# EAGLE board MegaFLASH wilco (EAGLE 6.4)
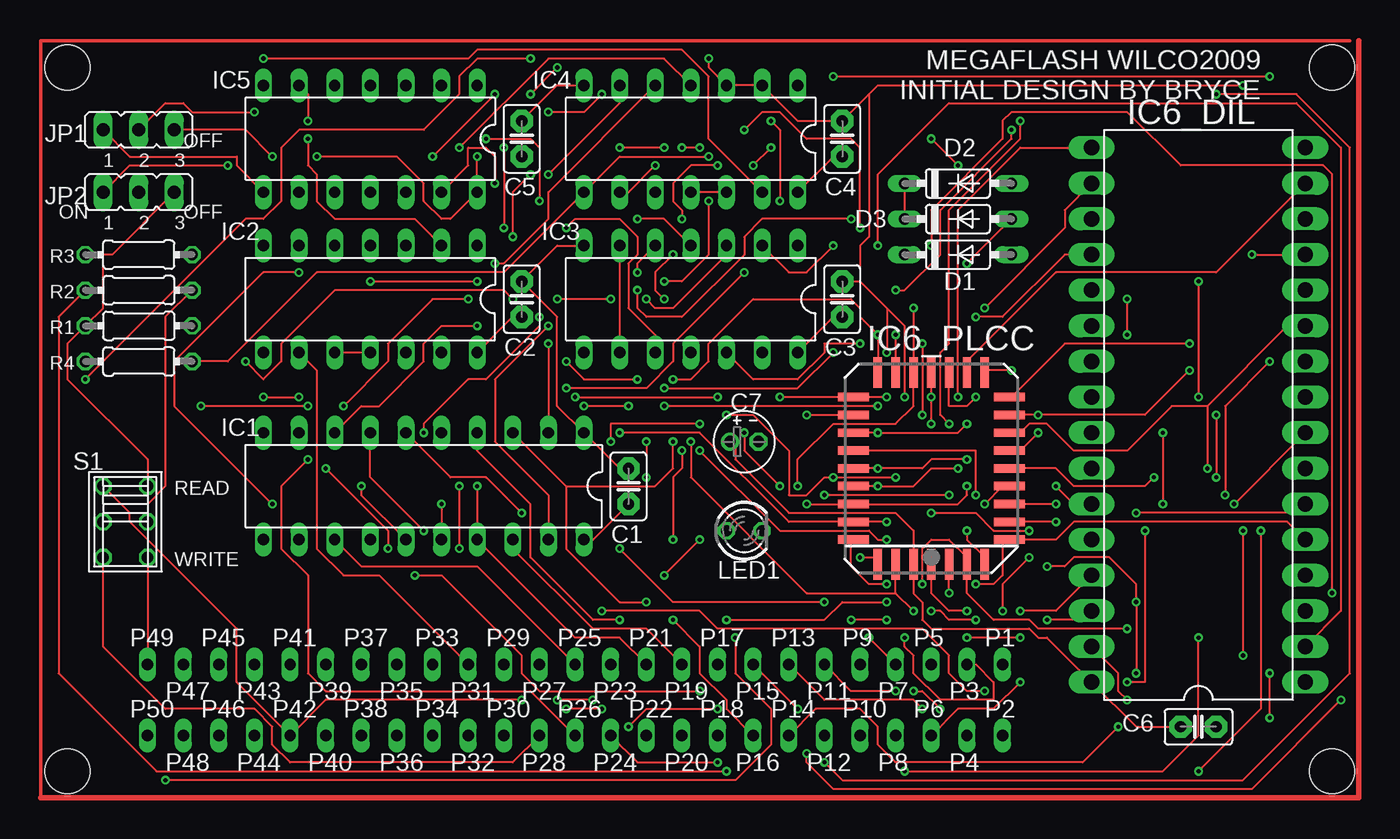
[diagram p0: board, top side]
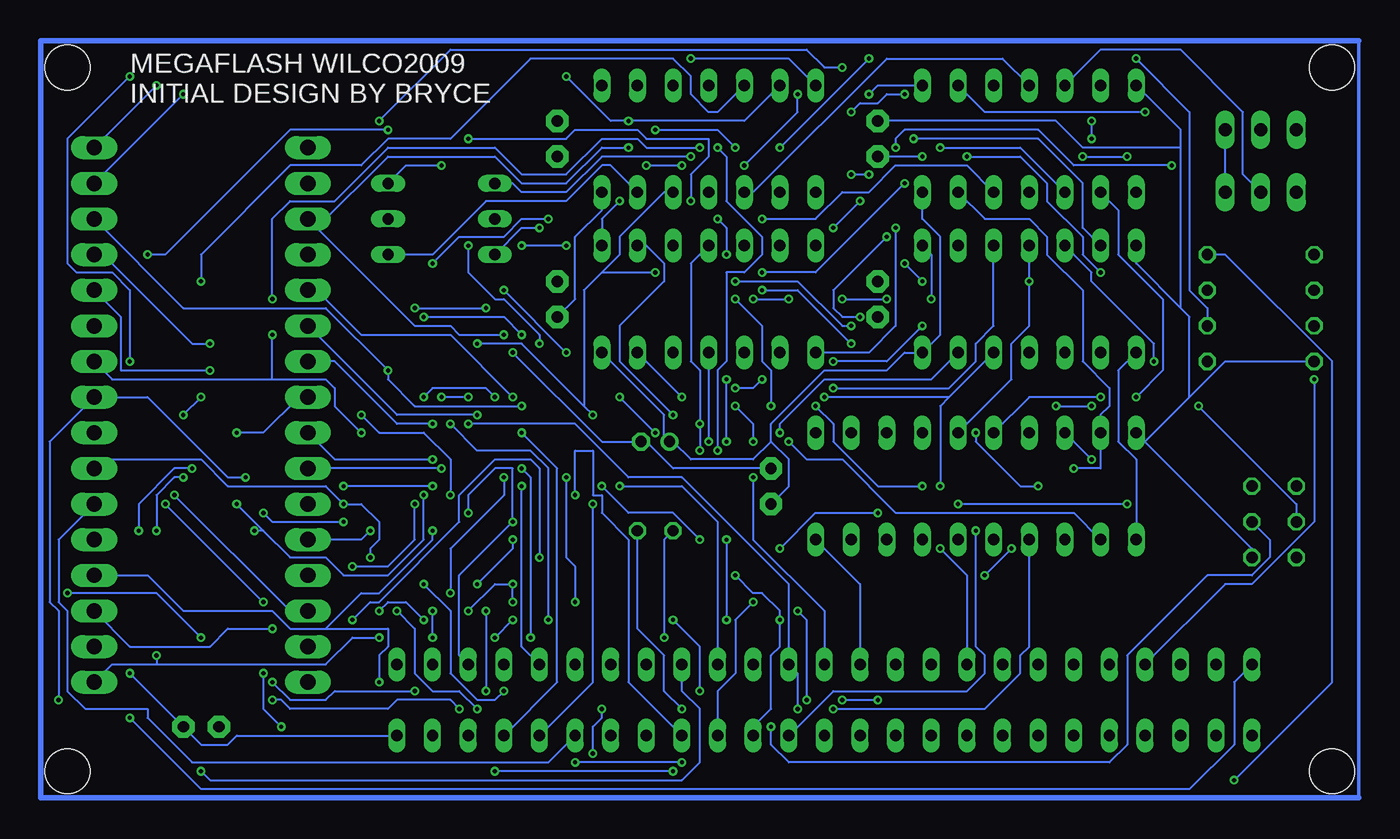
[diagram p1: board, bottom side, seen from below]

No outline drawn. Coordinates in mm, seen from the top.
Copper layers (1*2*15*16): Top 0.035mm / dielectric 0.2mm / Route2 0.0175mm / dielectric 1.1mm / Route15 0.0175mm / dielectric 0.2mm / Bottom 0.035mm
Design rules "SeeedStudio_DRU_no_angle_20130527": minimum track width 6mil, minimum drill 12mil, track to track 6mil, track to pad 6mil, pad to pad 6mil, via to via 6mil, smd to smd 0mil, copper to edge 10mil, drill to drill 10mil, minimum pad ring 6mil, minimum via ring 6mil, stop-mask expansion 2mil, vias tented up to drill 25mil, thermal gap 10mil
Holes 3.2 mm at 1.91,52.07 92.08,52.07 92.08,1.91 1.91,1.91

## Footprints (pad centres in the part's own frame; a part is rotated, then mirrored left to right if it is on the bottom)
C2.5-2 = drill 0.813 pad 1.6 octagon: 1 -1.27,0; 2 1.27,0
E2-4 = drill 0.813 pad 1.27: + -1.016,0 | drill 0.813 pad 1.27 octagon: - 1.016,0
DO35-7 = drill 0.813 long: A 3.81,0; C -3.81,0
CPC_BUS_EXP_BOTTOM = drill 0.813 long: 1 30.48,3.81; 2 30.48,-1.27; 3 27.94,3.81; 4 27.94,-1.27; 5 25.4,3.81; 6 25.4,-1.27; 7 22.86,3.81; 8 22.86,-1.27; 9 20.32,3.81; 10 20.32,-1.27; 11 17.78,3.81; 12 17.78,-1.27; 13 15.24,3.81; 14 15.24,-1.27; 15 12.7,3.81; 16 12.7,-1.27; 17 10.16,3.81; 18 10.16,-1.27; 19 7.62,3.81; 20 7.62,-1.27; 21 5.08,3.81; 22 5.08,-1.27; 23 2.54,3.81; 24 2.54,-1.27; 25 0,3.81; 26 0,-1.27; 27 -2.54,3.81; 28 -2.54,-1.27; 29 -5.08,3.81; 30 -5.08,-1.27; 31 -7.62,3.81; 32 -7.62,-1.27; 33 -10.16,3.81; 34 -10.16,-1.27; 35 -12.7,3.81; 36 -12.7,-1.27; 37 -15.24,3.81; 38 -15.24,-1.27; 39 -17.78,3.81; 40 -17.78,-1.27; 41 -20.32,3.81; 42 -20.32,-1.27; 43 -22.86,3.81; 44 -22.86,-1.27; 45 -25.4,3.81; 46 -25.4,-1.27; 47 -27.94,3.81; 48 -27.94,-1.27; 49 -30.48,3.81; 50 -30.48,-1.27
DIL20 = drill 0.813 long: 1 -11.43,-3.81; 2 -8.89,-3.81; 3 -6.35,-3.81; 4 -3.81,-3.81; 5 -1.27,-3.81; 6 1.27,-3.81; 7 3.81,-3.81; 8 6.35,-3.81; 9 8.89,-3.81; 10 11.43,-3.81; 11 11.43,3.81; 12 8.89,3.81; 13 6.35,3.81; 14 3.81,3.81; 15 1.27,3.81; 16 -1.27,3.81; 17 -3.81,3.81; 18 -6.35,3.81; 19 -8.89,3.81; 20 -11.43,3.81
DIL14 = drill 0.813 long: 1 -7.62,-3.81; 2 -5.08,-3.81; 3 -2.54,-3.81; 4 0,-3.81; 5 2.54,-3.81; 6 5.08,-3.81; 7 7.62,-3.81; 8 7.62,3.81; 9 5.08,3.81; 10 2.54,3.81; 11 0,3.81; 12 -2.54,3.81; 13 -5.08,3.81; 14 -7.62,3.81
DIL32 = drill 1.1 long: 1 -21.59,-8.89; 2 -19.05,-8.89; 3 -16.51,-8.89; 4 -13.97,-8.89; 5 -11.43,-8.89; 6 -8.89,-8.89; 7 -6.35,-8.89; 8 -3.81,-8.89; 9 -1.27,-8.89; 10 1.27,-8.89; 11 3.81,-8.89; 12 6.35,-8.89; 13 8.89,-8.89; 14 11.43,-8.89; 15 13.97,-8.89; 16 16.51,-8.89; 17 16.51,6.35; 18 13.97,6.35; 19 11.43,6.35; 20 8.89,6.35; 21 6.35,6.35; 22 3.81,6.35; 23 1.27,6.35; 24 -1.27,6.35; 25 -3.81,6.35; 26 -6.35,6.35; 27 -8.89,6.35; 28 -11.43,6.35; 29 -13.97,6.35; 30 -16.51,6.35; 31 -19.05,6.35; 32 -21.59,6.35
PLCC32 = smd 2.2 x 0.6: 1 -6.83,0; 2 -6.83,-1.27; 3 -6.83,-2.54; 4 -6.83,-3.81; 14 6.83,-3.81; 15 6.83,-2.54; 16 6.83,-1.27; 17 6.83,0; 18 6.83,1.27; 19 6.83,2.54; 20 6.83,3.81; 30 -6.83,3.81; 31 -6.83,2.54; 32 -6.83,1.27 | smd 0.6 x 2.2: 5 -5.08,-5.56; 6 -3.81,-5.56; 7 -2.54,-5.56; 8 -1.27,-5.56; 9 0,-5.56; 10 1.27,-5.56; 11 2.54,-5.56; 12 3.81,-5.56; 13 5.08,-5.56; 21 5.08,5.56; 22 3.81,5.56; 23 2.54,5.56; 24 1.27,5.56; 25 0,5.56; 26 -1.27,5.56; 27 -2.54,5.56; 28 -3.81,5.56; 29 -5.08,5.56
JP2 = drill 0.914 long: 1 -2.54,0; 2 0,0; 3 2.54,0
LED3MM = drill 0.813 octagon: A -1.27,0; K 1.27,0
0204/7 = drill 0.813 octagon: 1 -3.81,0; 2 3.81,0
2P2T-FINO = drill 0.813 octagon: 1 -2.54,-1.27; 2 0,-1.27; 3 2.54,-1.27; 4 -2.54,1.905; 5 0,1.905; 6 2.54,1.905

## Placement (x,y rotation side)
C1  100nF  [C2.5-2]  41.91,22.23 90 top
C2  100nF  [C2.5-2]  34.29,35.56 90 top
C3  100nF  [C2.5-2]  57.15,35.56 90 top
C4  100nF  [C2.5-2]  57.15,46.99 90 top
C5  100nF  [C2.5-2]  34.29,46.99 90 top
C6  100nF  [C2.5-2]  82.55,5.08 0 top
C7  100microF  [E2-4]  50.16,25.4 0 top
D1  1N4148DO35-7  [DO35-7]  65.41,38.73 0 top
D2  1N4148DO35-7  [DO35-7]  65.41,43.81 0 top
D3  1N4148DO35-7  [DO35-7]  65.41,41.27 0 top
EC1  CPC_BUS_EXPBOTTOM  [CPC_BUS_EXP_BOTTOM]  38.1,5.71 0 top
IC1  74LS374N  [DIL20]  27.3,22.23 180 top
IC2  74LS32N  [DIL14]  23.5,35.56 180 top
IC3  74LS32N  [DIL14]  46.35,35.56 180 top
IC4  74LS02N  [DIL14]  46.35,46.99 180 top
IC5  74LS20N  [DIL14]  23.5,46.99 180 top
IC6_DIL  29C040DIL32  [DIL32]  81.28,29.84 90 top
IC6_PLCC  29C040PLCC32  [PLCC32]  63.5,23.5 90 top
JP1  ROM 7  [JP2]  6.99,47.62 0 top
JP2  ROM 0  [JP2]  6.99,43.18 0 top
LED1  TLLR4400  [LED3MM]  50.16,19.05 0 top
R1  1K  [0204/7]  6.99,33.66 180 top
R2  220R  [0204/7]  6.99,36.2 180 top
R3  1K  [0204/7]  6.99,38.73 0 top
R4  1K  [0204/7]  6.99,31.11 0 top
S1  DPDT  [2P2T-FINO]  5.71,19.68 270 top

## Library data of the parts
C1-C6 = capacitor-wima
C7 = resistor
D1-D3 = diode
EC1 IC6_DIL IC6_PLCC S1 = Mio
IC1-IC5 = 74xx-eu
JP1 JP2 = jumper
LED1 = led; MF: VISHAY SEMICONDUCTOR; OC_FARNELL: 1612437
R1-R4 = eagle-ltspice; SPICEMODEL: NONE; SPICEPREFIX: R

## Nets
GND: C1.2 C2.2 C3.2 C4.2 C5.2 C6.2 C7.- EC1.2 EC1.49 IC1.1 IC1.10 IC2.7 IC3.7 IC4.2 IC4.3 IC4.7 IC5.7 IC6_DIL.16 IC6_PLCC.16 R4.1 S1.6
N$1: EC1.3 IC5.1
N$2: EC1.12 IC6_DIL.6 IC6_PLCC.6
N$3: EC1.31 IC2.9
N$5: EC1.7 IC6_DIL.25 IC6_PLCC.25
N$6: IC1.9 IC3.5 IC5.13 IC6_DIL.29 IC6_PLCC.29
N$7: IC1.12 IC3.4 IC5.12 IC6_DIL.3 IC6_PLCC.3
N$8: EC1.9 IC6_DIL.26 IC6_PLCC.26
N$9: EC1.11 IC6_DIL.5 IC6_PLCC.5
N$10: EC1.13 IC6_DIL.7 IC6_PLCC.7
N$11: EC1.15 IC6_DIL.9 IC6_PLCC.9
N$12: EC1.17 IC6_DIL.11 IC6_PLCC.11
N$13: IC1.6 IC3.2 IC5.9 IC6_DIL.2 IC6_PLCC.2
N$14: EC1.6 IC6_DIL.4 IC6_PLCC.4
N$15: EC1.8 IC6_DIL.23 IC6_PLCC.23
N$16: EC1.10 IC6_DIL.27 IC6_PLCC.27
N$17: EC1.14 IC6_DIL.8 IC6_PLCC.8
N$18: EC1.16 IC6_DIL.10 IC6_PLCC.10
N$19: EC1.18 IC6_DIL.12 IC6_PLCC.12
N$20: EC1.26 IC1.8 IC6_DIL.13 IC6_PLCC.13
N$21: EC1.24 IC1.7 IC6_DIL.15 IC6_PLCC.15
N$22: EC1.22 IC1.4 IC6_DIL.18 IC6_PLCC.18
N$23: EC1.20 IC1.3 IC6_DIL.20 IC6_PLCC.20
N$24: EC1.25 IC1.13 IC6_DIL.14 IC6_PLCC.14
N$25: EC1.23 IC1.14 IC6_DIL.17 IC6_PLCC.17
N$26: EC1.21 IC1.17 IC6_DIL.19 IC6_PLCC.19
N$27: EC1.19 IC1.18 IC6_DIL.21 IC6_PLCC.21
N$28: IC1.15 IC3.1 IC4.6 IC6_DIL.30 IC6_PLCC.30
N$29: IC1.5 IC2.4 IC4.5 IC6_DIL.1 IC6_PLCC.1
N$30: IC2.3 IC4.11 IC4.12 IC6_DIL.22 IC6_PLCC.22
N$33: EC1.42 IC6_DIL.24 IC6_PLCC.24 S1.1
N$34: IC3.11 IC6_DIL.31 IC6_PLCC.31
N$35: D1.C EC1.43
N$36: EC1.28 S1.3
N$37: D1.A IC4.13 R1.1
N$38: LED1.A R3.2
N$39: LED1.K R2.1 S1.5
N$40: IC3.12 R2.2
N$41: IC2.5 IC3.3
N$42: EC1.33 IC2.12 IC3.13
N$43: IC3.6 IC3.9
N$44: IC2.6 IC3.10
N$45: IC1.11 IC2.8
N$46: IC2.1 S1.2
N$47: IC2.2 IC5.6
N$48: IC2.10 IC2.11
N$49: IC4.4 IC5.10
N$50: IC4.10 IC5.4
N$51: IC5.8 JP1.1
N$52: IC5.5 JP2.2
N$53: IC5.2 JP1.2
N$54: IC3.8 JP2.1
N$55: D2.A IC1.19
N$56: IC1.16 IC4.9
N$57: D2.C D3.C IC4.8 R4.2
N$58: EC1.5 IC2.13 IC6_DIL.28 IC6_PLCC.28
N$59: D3.A IC1.2
VCC: C1.1 C2.1 C3.1 C4.1 C5.1 C6.1 C7.+ EC1.27 IC1.20 IC2.14 IC3.14 IC4.14 IC5.14 IC6_DIL.32 IC6_PLCC.32 JP1.3 JP2.3 R1.2 R3.1 S1.4

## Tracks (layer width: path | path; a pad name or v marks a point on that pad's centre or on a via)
GND  (via drill 0.3)
  Top 0.152: IC3.7 36.83,39.37 C2.2 36.83,34.29 36.83,27.94 IC1.1 41.27,23.5 C1.2 | IC6_PLCC.16 64.77,27.94 66.04,27.94 v66.67,28.57 | v61.59,28.57 61.59,33.66 60.33,34.92 | 58.42,36.83 60.33,34.92 | C3.2 58.42,36.83 | v85.72,50.8 59.69,50.8 59.05,50.16 | 59.05,50.16 C4.2 53.98,48.26 IC4.2 IC4.3 47.62,52.07 v47.62,52.7 | 58.42,36.83 58.42,39.37 59.05,40.01 59.05,50.16 | 60.33,34.92 v60.33,31.75 | IC4.7 36.83,50.8 C5.2 | S1.6 EC1.49 | v87.63,5.71 v87.63,8.89
  Bottom 0.152: C1.2 48.9,23.5 50.8,25.4 C7.- 53.98,25.4 v60.33,31.75 | v66.67,28.57 66.04,29.21 62.23,29.21 v61.59,28.57 | v85.72,50.8 IC6_DIL.16 | EC1.2 80.01,4.45 80.64,3.81 82.55,3.81 C6.2 v87.63,8.89 | 15.24,25.4 7.62,17.78 S1.6 | 15.24,25.4 IC1.10 | R4.1 9.53,31.11 12.06,28.57 | 15.24,25.4 12.06,28.57 | IC2.7 15.88,38.1 12.7,34.92 | 12.7,34.92 12.06,34.29 12.06,28.57 | IC5.7 12.7,47.62 12.7,46.35 | 12.7,34.92 12.7,46.35 | C5.2 21.59,48.26 19.68,46.35 12.7,46.35 | v87.63,5.71 82.55,0.64 12.06,0.64 8.89,3.81 8.89,8.26 EC1.49 | v47.62,52.7 40.64,52.7 IC4.7
N$1  (via drill 0.3)
  Top 0.152: v36.83,52.07 v34.92,50.16 | v69.85,48.26 69.85,46.99 64.77,41.91 64.77,32.38 64.14,31.75 64.14,27.3 v64.77,26.67 | v60.33,12.7 v57.78,12.7 | v61.59,11.43 61.59,10.79 62.23,10.16 62.23,8.89 64.14,6.99 67.94,6.99 67.94,8.26 66.67,9.53 EC1.3
  Bottom 0.152: IC5.1 34.29,50.8 v34.92,50.16 | v36.83,52.07 38.1,52.07 39.37,53.34 64.77,53.34 v69.85,48.26 | v64.77,26.67 62.87,24.77 59.05,24.77 57.78,23.5 v57.78,12.7 | v61.59,11.43 v60.33,12.7
N$2  (via drill 0.3)
  Top 0.152: v72.39,19.68 IC6_PLCC.6 | v78.11,20.32 89.53,20.32 IC6_DIL.6
  Bottom 0.152: v72.39,19.68 77.47,19.68 v78.11,20.32 | EC1.12 57.78,2.54 83.19,2.54 86.36,5.71 86.36,6.35 90.81,6.35 92.08,7.62 92.08,13.34 92.71,13.97 92.71,18.41 IC6_DIL.6
N$3
  Top 0.152: EC1.31 24.13,15.88 21.59,15.88 19.68,17.78 19.68,30.48 IC2.9
N$5  (via drill 0.3)
  Top 0.152: IC6_PLCC.25 v59.69,23.5 62.87,23.5 63.5,24.13 v66.04,24.13 | v59.05,11.43 EC1.7
  Bottom 0.152: v66.04,24.13 73.03,24.13 IC6_DIL.25 | v59.05,11.43 59.05,22.86 v59.69,23.5
N$6  (via drill 0.3)
  Top 0.152: v60.33,15.24 59.05,15.24 57.78,16.51 57.78,18.41 IC6_PLCC.29 | v63.5,13.34 64.14,13.34 64.77,12.7 v66.67,12.7 | v69.85,13.34 72.39,13.34 IC6_DIL.29 | IC3.5 42.55,38.1 v42.55,37.47 | v32.38,43.81 32.38,45.72 31.75,46.35 30.48,46.35 30.48,45.09 IC5.13 | v60.33,13.97 57.15,13.97 55.88,12.7 v48.9,12.7 | v46.99,7.62 35.56,7.62 34.29,8.89 34.29,10.16 28.57,15.88 v26.67,15.88 | v24.77,17.78 24.77,19.05 v20.32,23.5
  Bottom 0.152: v63.5,13.34 61.59,15.24 v60.33,15.24 v60.33,13.97 | v66.67,12.7 67.94,13.97 69.22,13.97 v69.85,13.34 | IC5.13 26.67,41.27 23.5,41.27 22.23,40.01 22.23,38.73 19.68,36.2 19.68,31.11 17.78,29.21 17.78,27.94 18.41,27.3 IC1.9 18.41,23.5 v20.32,23.5 | v42.55,37.47 38.73,37.47 v32.38,43.81 | v48.9,12.7 46.99,10.79 v46.99,7.62 | v24.77,17.78 v26.67,15.88
N$7  (via drill 0.3)
  Top 0.152: v77.47,12.06 71.12,12.06 70.48,12.7 67.94,12.7 66.04,14.61 IC6_PLCC.3 66.04,17.14 64.77,18.41 63.5,18.41 62.87,17.78 v62.87,15.24 | v40.64,25.4 40.64,26.67 v46.99,26.67 | v42.55,41.27 44.45,41.27 IC3.4 | v60.33,18.41 59.69,18.41 59.05,19.05 52.7,19.05 v46.99,24.77
  Bottom 0.152: v77.47,12.06 80.64,12.06 81.92,10.79 87.63,10.79 IC6_DIL.3 | IC1.12 20.32,20.32 33.02,20.32 36.83,24.13 39.37,24.13 v40.64,25.4 | IC3.4 47.62,38.1 47.62,31.11 46.99,30.48 v46.99,26.67 v46.99,24.77 | IC5.12 27.94,45.09 33.02,45.09 34.92,43.18 36.83,43.18 38.73,41.27 v42.55,41.27 | v62.87,15.24 60.33,17.78 v60.33,18.41
N$8  (via drill 0.3)
  Top 0.152: IC6_PLCC.26 v59.69,22.23 62.23,22.23 63.5,23.5 v65.41,23.5
  Bottom 0.152: v59.69,22.23 59.69,10.79 EC1.9 | v65.41,23.5 IC6_DIL.26
N$9  (via drill 0.3)
  Top 0.152: IC6_DIL.5 88.9,19.68 73.66,19.68 72.39,18.41 IC6_PLCC.5 68.58,18.41 68.58,15.88 67.94,15.24 v66.67,15.24 | EC1.11 57.78,7.62 v60.96,7.62
  Bottom 0.152: v60.96,7.62 61.59,6.99 62.87,6.99 64.77,8.89 64.77,13.34 v66.67,15.24
N$10  (via drill 0.3)
  Top 0.152: v72.39,20.95 IC6_PLCC.7 | EC1.13 55.88,6.99 62.23,6.99 v62.87,6.35 | v68.58,13.34 68.58,15.24 v70.48,17.14
  Bottom 0.152: IC6_DIL.7 89.53,24.13 82.55,24.13 80.64,22.23 73.66,22.23 v72.39,20.95 71.12,20.95 69.85,19.68 69.85,18.41 70.48,17.78 v70.48,17.14 | v62.87,6.35 64.14,7.62 66.04,7.62 67.31,8.89 67.31,12.06 v68.58,13.34
N$11  (via drill 0.3)
  Top 0.152: IC6_PLCC.9 72.39,23.5 73.66,22.23 78.74,22.23 v79.38,22.86 | v53.98,6.35 EC1.15 | v54.61,3.17 54.61,2.54 56.52,0.64 86.36,0.64 v92.71,6.99
  Bottom 0.152: v79.38,22.86 80.64,22.86 86.36,28.57 IC6_DIL.9 93.34,25.4 93.34,13.97 92.71,13.34 v92.71,6.99 | v53.98,6.35 53.98,5.71 54.61,5.08 v54.61,3.17
N$12  (via drill 0.3)
  Top 0.152: IC6_PLCC.11 69.85,26.04 70.48,26.67 71.75,26.67 73.66,24.77 77.47,24.77 80.64,27.94 83.19,27.94 | 83.19,27.94 88.9,33.66 IC6_DIL.11 | v82.55,1.91 87,6.35 v87,19.05 | 83.19,27.94 v83.19,23.5
  Bottom 0.152: EC1.17 48.26,7.62 46.99,6.35 46.99,2.54 48.26,1.27 81.92,1.27 v82.55,1.91 | v87,19.05 87,20.95 84.45,23.5 v83.19,23.5
N$13  (via drill 0.3)
  Top 0.152: v15.88,28.57 v18.41,28.57 | v64.77,14.61 IC6_PLCC.2 | v60.96,22.86 v56.52,22.86 55.88,22.86 54.61,21.59 53.34,21.59 53.34,24.77 50.8,27.3 v48.9,27.3 | IC6_DIL.2 92.71,13.34 92.71,46.35 89.53,49.53 64.77,49.53 59.69,44.45 v59.69,39.37 | v56.52,39.37 54.61,37.47 53.34,37.47 IC3.2 | IC1.6 29.21,22.86 31.75,22.86 v34.29,20.32 | v41.27,17.78 45.09,13.97 v55.88,13.97
  Bottom 0.152: IC1.6 23.5,28.57 v18.41,28.57 | v15.88,28.57 13.97,30.48 13.97,35.56 17.14,38.73 17.14,41.91 IC5.9 | v64.77,14.61 64.77,17.78 60.96,21.59 v60.96,22.86 | v48.9,27.3 52.7,31.11 52.7,33.66 49.53,36.83 49.53,38.1 50.8,39.37 IC3.2 | v56.52,39.37 v59.69,39.37 | v34.29,20.32 38.73,20.32 v41.27,17.78 | v55.88,13.97 55.88,16.51 56.52,17.14 v56.52,22.86
N$14  (via drill 0.3)
  Top 0.152: v66.04,19.05 66.04,18.41 67.31,17.14 IC6_PLCC.4 | EC1.6 65.41,6.35 67.94,6.35 v69.85,8.26
  Bottom 0.152: v66.04,19.05 66.04,18.41 69.85,14.61 71.12,14.61 73.66,12.06 | 73.66,12.06 76.2,12.06 77.47,13.34 83.82,13.34 86.36,15.88 IC6_DIL.4 | v69.85,8.26 69.85,10.16 69.22,10.79 69.22,12.06 73.66,12.06
N$15  (via drill 0.3)
  Top 0.152: IC6_PLCC.23 v59.69,26.04 65.41,26.04 v66.04,26.67
  Bottom 0.152: v59.69,26.04 57.15,23.5 57.15,8.26 EC1.8 | IC6_DIL.23 73.03,31.11 68.58,26.67 v66.04,26.67
N$16  (via drill 0.3)
  Top 0.152: v54.61,20.95 IC6_PLCC.27 65.41,20.95 66.04,21.59 v66.04,22.23 | IC6_DIL.27 73.66,20.95 v72.39,22.23
  Bottom 0.152: v54.61,20.95 54.61,8.26 EC1.10 | v66.04,22.23 v72.39,22.23
N$17  (via drill 0.3)
  Top 0.152: v67.31,20.95 68.58,22.23 IC6_PLCC.8 | v71.75,16.51 73.03,16.51 73.66,17.14 76.2,17.14 78.11,15.24 v78.11,13.97 v78.11,8.89 | IC6_DIL.8 v85.09,20.95 | EC1.14 55.24,6.35 58.42,6.35 59.69,5.08 59.69,3.81 60.96,2.54 74.3,2.54 v76.83,5.08
  Bottom 0.152: v67.31,20.95 67.31,18.41 69.22,16.51 v71.75,16.51 | v85.09,20.95 v78.11,13.97 | v76.83,5.08 78.11,6.35 v78.11,8.89
N$18  (via drill 0.3)
  Top 0.152: IC6_PLCC.10 69.85,24.77 v71.12,26.04 | EC1.16 48.9,6.35 48.9,6.99 46.99,8.89 46.99,10.79 v45.09,12.7 | v45.09,18.41 45.09,22.86 45.72,23.5 v45.72,24.77 | v46.99,46.35 v45.72,46.35 | v77.47,33.02 v77.47,35.56
  Bottom 0.152: v71.12,26.04 73.03,27.94 73.03,29.21 73.66,29.84 77.47,29.84 | 77.47,29.84 88.9,29.84 IC6_DIL.10 | v45.09,18.41 v45.09,12.7 | v45.72,24.77 45.72,30.48 45.09,31.11 45.09,37.47 43.81,37.47 42.55,38.73 42.55,40.01 45.09,42.55 45.09,45.72 v45.72,46.35 | v46.99,46.35 50.8,46.35 51.44,46.99 53.98,46.99 56.52,44.45 59.69,44.45 61.59,46.35 69.22,46.35 73.03,42.55 76.2,42.55 77.47,41.27 v77.47,35.56 | 77.47,29.84 v77.47,33.02
N$19  (via drill 0.3)
  Top 0.152: IC6_PLCC.12 v71.12,27.3 78.74,27.3 v81.92,30.48 | v64.77,21.59 v55.88,21.59
  Bottom 0.152: v81.92,30.48 88.27,30.48 88.27,34.29 IC6_DIL.12 | EC1.18 52.07,8.26 52.07,18.41 53.98,20.32 53.98,21.59 54.61,21.59 54.61,24.77 55.88,24.77 v55.88,21.59 | v64.77,21.59 64.77,24.13 66.67,26.04 69.85,26.04 v71.12,27.3
N$20  (via drill 0.3)
  Top 0.152: v81.92,32.38 73.03,32.38 69.22,28.57 IC6_PLCC.13 | EC1.26 34.92,7.62 20.32,7.62 19.05,8.89 19.05,15.88 17.14,17.78 17.14,22.23 v19.05,24.13 | v86.36,38.73 IC6_DIL.13 | v69.22,47.62 69.22,46.99 64.14,41.91 64.14,38.73 61.59,36.2 v60.96,36.2 | v56.52,31.75 53.98,29.21 v44.45,29.21 | v42.55,29.84 38.73,29.84 v37.47,31.11 | v31.11,33.66 28.57,33.66 27.3,32.38 27.3,31.11 24.13,27.94 22.86,27.94 IC1.8
  Bottom 0.152: v81.92,32.38 83.19,32.38 89.53,38.73 IC6_DIL.13 | IC1.8 v19.05,24.13 | v86.36,38.73 85.09,38.73 76.2,47.62 v69.22,47.62 | v56.52,31.75 v60.96,36.2 | v44.45,29.21 43.18,29.21 v42.55,29.84 | v37.47,31.11 33.66,31.11 v31.11,33.66
N$21  (via drill 0.3)
  Top 0.152: IC6_PLCC.15 66.04,31.11 72.39,37.47 83.82,37.47 IC6_DIL.15 | IC1.7 23.5,22.86 v27.3,19.05 | v83.82,50.16 89.53,50.16 93.34,46.35 93.34,8.89 85.72,1.27 57.15,1.27 v55.88,2.54 | v48.26,2.54 42.55,2.54 EC1.24
  Bottom 0.152: v27.3,19.05 27.3,10.79 26.67,10.16 26.67,8.89 27.94,7.62 37.47,7.62 EC1.24 | v83.82,50.16 IC6_DIL.15 | v48.26,2.54 v55.88,2.54
N$22  (via drill 0.3)
  Top 0.152: v62.23,34.92 IC6_PLCC.18 62.23,27.94 60.96,26.67 56.52,26.67 53.98,24.13 v53.98,22.23 | v67.31,34.92 73.03,40.64 73.03,41.91 IC6_DIL.18 | IC1.4 31.11,24.77 34.92,20.95 34.92,17.14 39.37,12.7 v41.27,12.7 | v44.45,15.88 v46.99,18.41
  Bottom 0.152: v67.31,34.92 v62.23,34.92 | EC1.22 43.18,5.08 41.91,6.35 41.91,10.16 41.27,10.79 v41.27,12.7 41.27,13.34 42.55,14.61 43.18,14.61 v44.45,15.88 | v53.98,22.23 52.07,20.32 48.9,20.32 v46.99,18.41
N$23  (via drill 0.3)
  Top 0.152: IC6_PLCC.20 v59.69,33.02 58.42,34.29 58.42,34.92 57.78,35.56 50.8,35.56 47.62,32.38 47.62,31.11 46.35,29.84 v45.09,29.84 | v66.67,34.29 68.58,34.29 73.03,38.73 IC6_DIL.20 | v43.18,13.97 41.27,13.97 37.47,17.78 37.47,22.23 | IC1.3 37.47,22.23 | v45.09,25.4 45.09,23.5 43.81,22.23 37.47,22.23
  Bottom 0.152: v59.69,33.02 60.96,34.29 v66.67,34.29 | EC1.20 45.72,7.62 44.45,8.89 44.45,12.7 v43.18,13.97 | v45.09,25.4 v45.09,29.84
N$24  (via drill 0.3)
  Top 0.152: EC1.25 31.11,16.51 22.86,16.51 IC1.13 | v69.22,30.48 67.31,30.48 IC6_PLCC.14 | v43.18,25.4 v43.18,22.86 | v59.69,27.94 v44.45,27.94
  Bottom 0.152: IC6_DIL.14 83.82,34.92 73.66,34.92 v69.22,30.48 69.22,29.84 67.31,27.94 v59.69,27.94 | EC1.25 38.1,13.34 43.18,18.41 v43.18,22.86 | v43.18,25.4 43.18,26.67 v44.45,27.94
N$25  (via drill 0.3)
  Top 0.152: v63.5,26.67 v63.5,28.57 IC6_PLCC.17 | v40.01,6.35 v37.47,6.35 | IC6_DIL.17 69.85,46.35 65.41,41.91 v65.41,28.57
  Bottom 0.152: v63.5,26.67 55.88,26.67 52.07,22.86 48.26,22.86 40.64,15.24 EC1.23 40.01,8.89 v40.01,6.35 | IC1.14 23.5,10.79 24.13,10.16 24.13,8.89 26.67,6.35 v37.47,6.35 | v63.5,28.57 v65.41,28.57
N$26  (via drill 0.3)
  Top 0.152: EC1.21 41.27,11.43 38.1,11.43 IC1.17 v31.11,22.23 | v60.96,33.02 IC6_PLCC.19 | v41.91,27.94 v38.73,27.94 | v44.45,35.56 43.81,36.2 43.81,37.47 v45.09,38.73 | v45.72,41.27 45.72,41.91 45.09,42.55 45.09,43.81 46.35,45.09 v48.26,45.09 | v52.07,46.35 v50.8,45.09
  Bottom 0.152: v60.96,33.02 64.14,33.02 64.77,33.66 67.31,33.66 74.3,40.64 | v31.11,22.23 34.29,22.23 37.47,25.4 37.47,26.67 v38.73,27.94 | v41.91,27.94 41.91,30.48 42.55,31.11 42.55,33.66 v44.45,35.56 | v45.09,38.73 45.09,40.64 v45.72,41.27 | v50.8,45.09 v48.26,45.09 | v52.07,46.35 53.98,46.35 56.52,43.81 59.69,43.81 61.59,45.72 69.22,45.72 74.3,40.64 | 74.3,40.64 IC6_DIL.19
N$27  (via drill 0.3)
  Top 0.152: IC1.18 33.66,17.78 39.37,12.06 43.18,12.06 EC1.19 | v60.33,28.57 IC6_PLCC.21 v52.7,28.57 | v52.7,22.23 50.16,24.77 v50.16,26.04
  Bottom 0.152: v60.33,28.57 64.77,33.02 71.12,33.02 74.3,36.2 IC6_DIL.21 | EC1.19 45.72,19.68 48.26,22.23 v52.7,22.23 | v52.7,28.57 v50.16,26.04
N$28  (via drill 0.3)
  Top 0.152: v58.42,17.14 59.69,17.14 IC6_PLCC.30 | v71.75,12.7 74.3,12.7 IC6_DIL.30 | IC1.15 22.86,21.59 v22.86,22.23 | v27.3,26.04 27.3,26.67 30.48,29.84 31.75,29.84 35.56,33.66 v35.56,34.29 | v33.66,40.01 33.66,43.18 v34.92,44.45 | v36.2,44.45 41.27,49.53 IC4.6 | v52.7,42.55 52.7,47.62 v52.07,48.26 | v84.45,21.59 84.45,27.94 v87.63,31.11 | v56.52,51.44 v87.63,51.44
  Bottom 0.152: v58.42,17.14 58.42,23.5 59.05,24.13 61.59,24.13 64.14,21.59 64.14,19.68 69.85,13.97 70.48,13.97 v71.75,12.7 | v22.86,22.23 24.13,22.23 27.3,25.4 v27.3,26.04 | v35.56,34.29 36.83,34.29 37.47,34.92 37.47,36.2 v33.66,40.01 | v36.2,44.45 v34.92,44.45 | IC3.1 53.98,41.27 v52.7,42.55 | IC4.6 43.81,48.26 v52.07,48.26 53.34,48.26 v56.52,51.44 | IC6_DIL.30 76.2,13.34 v84.45,21.59 | v87.63,31.11 87.63,36.2 88.9,37.47 91.44,37.47 92.08,38.1 92.08,46.99 v87.63,51.44
N$29  (via drill 0.3)
  Top 0.152: IC6_PLCC.1 63.5,14.61 64.77,13.34 v66.04,13.34 | v69.85,11.43 v66.04,11.43 | IC4.5 36.2,43.18 36.2,41.27 33.02,38.1 v32.38,38.1 | v23.5,36.83 v31.11,36.83 | v85.72,19.05 v85.72,10.16 | v83.82,27.3 v83.82,22.86 | v82.55,36.83 v82.55,28.57
  Bottom 0.152: v66.04,11.43 v66.04,13.34 | v69.85,11.43 71.75,11.43 73.66,9.53 85.72,9.53 | 85.72,9.53 88.9,9.53 IC6_DIL.1 | IC2.4 v23.5,36.83 23.5,33.66 24.77,32.38 24.77,29.84 IC1.5 | v31.11,36.83 v32.38,38.1 | v85.72,10.16 85.72,9.53 | v85.72,19.05 85.72,21.59 84.45,22.86 v83.82,22.86 | v82.55,28.57 v83.82,27.3 | v82.55,36.83 82.55,38.73 76.2,45.09 71.12,45.09 69.22,46.99 64.77,46.99 59.05,52.7 48.9,52.7 47.62,51.44 47.62,50.16 46.35,48.9 45.72,48.9 IC4.5
N$30  (via drill 0.3)
  Top 0.152: v54.61,27.3 IC6_PLCC.22 | v37.47,29.21 43.18,29.21 45.09,31.11 45.09,32.38 v50.16,37.47 | IC4.12 IC4.11 | v62.87,32.38 v62.87,27.3
  Bottom 0.152: 55.24,27.94 v54.61,27.3 | 55.24,27.94 55.24,36.2 53.98,37.47 | 53.98,37.47 52.7,38.73 52.7,40.01 49.53,43.18 IC4.12 | IC2.3 26.04,33.66 27.3,32.38 27.3,31.11 29.21,29.21 v37.47,29.21 | 53.98,37.47 v50.16,37.47 | IC6_DIL.22 68.58,27.3 v62.87,27.3 | v62.87,32.38 59.69,32.38 55.24,27.94
N$31
  Bottom 0.254: 0,0 0,53.98
  Bottom 0.406: 0,53.98 93.98,53.98 93.98,0 0,0
N$32
  Top 0.254: 93.34,53.98 0,53.98 0,0
  Top 0.406: 0,0 93.98,0 93.98,53.98
N$33  (via drill 0.3)
  Top 0.152: S1.1 6.35,20.32 6.35,19.68 13.97,12.06 13.97,8.26 EC1.42 20.32,6.99 v34.29,6.99 | IC6_PLCC.24 66.67,24.77 v66.67,21.59 | v80.01,26.04 v80.01,20.95 | v39.37,6.99 v36.83,6.99 | v40.01,13.34 46.99,13.34 48.26,12.06 62.87,12.06 64.77,10.16 64.77,8.89 66.04,7.62 v67.31,7.62 | v77.47,8.26 78.74,8.26 v78.74,19.05
  Bottom 0.152: v66.67,21.59 66.67,18.41 69.22,15.88 72.39,15.88 73.66,17.14 76.2,17.14 78.11,19.05 | v80.01,20.95 78.11,19.05 | v80.01,26.04 78.11,26.04 75.56,28.57 IC6_DIL.24 | v36.83,6.99 v34.29,6.99 | v39.37,6.99 39.37,12.7 v40.01,13.34 | v67.31,7.62 73.03,7.62 73.66,6.99 76.2,6.99 v77.47,8.26 | 78.11,19.05 v78.74,19.05
N$34  (via drill 0.3)
  Top 0.152: 60.96,14.61 IC6_PLCC.31 | 60.96,14.61 54.61,14.61 46.35,22.86 v46.35,25.4 | IC6_DIL.31 76.83,8.89 76.83,7.62 v77.47,6.99 | v64.14,6.35 62.87,7.62 v62.23,7.62 | 60.96,14.61 v62.23,13.34
  Bottom 0.152: IC3.11 v46.35,25.4 | v77.47,6.99 76.83,6.99 76.2,6.35 69.22,6.35 68.58,6.99 64.77,6.99 v64.14,6.35 | v62.23,13.34 v62.23,7.62
N$35  (via drill 0.3)
  Top 0.152: v3.17,29.84 14.61,41.27 15.88,41.27 17.14,42.55 17.14,46.35 18.41,47.62 27.3,47.62 29.84,50.16 29.84,51.44 31.11,52.7 v34.92,52.7 | v44.45,46.35 v41.27,46.35 | v50.16,47.62 51.44,48.9 52.7,48.9 54.61,46.99 57.78,46.99 58.42,46.35 v58.42,40.64
  Bottom 0.152: EC1.43 9.53,15.24 7.62,15.24 3.17,19.68 v3.17,29.84 | v41.27,46.35 v34.92,52.7 | v44.45,46.35 45.72,47.62 v50.16,47.62 | v58.42,40.64 59.69,40.64 D1.C
N$36
  Top 0.152: S1.3 4.45,10.79 8.89,6.35 15.24,6.35 16.51,5.08 16.51,3.81 17.78,2.54 33.66,2.54 EC1.28
N$37  (via drill 0.3)
  Top 0.152: v15.88,52.7 30.48,52.7 31.11,53.34 45.72,53.34 47.62,51.44 47.62,46.99 IC4.13
  Bottom 0.152: R1.1 10.79,34.92 12.06,36.2 12.06,48.9 v15.88,52.7 | D1.A 66.04,38.73 62.23,42.55 56.52,42.55 53.98,45.09 53.34,45.09 IC4.13
N$38  (via drill 0.3)
  Top 0.152: v8.89,1.27 49.53,1.27 52.07,3.81 52.07,6.35 49.53,8.89 v49.53,11.43
  Bottom 0.152: R3.2 9.53,38.73 1.91,31.11 1.91,8.26 v8.89,1.27 | v49.53,11.43 49.53,18.41 LED1.A
N$39  (via drill 0.3)
  Top 0.152: S1.5 7.62,20.95 8.89,22.23 8.89,34.29 R2.1 | v48.26,6.35 43.18,6.35 v41.91,5.08
  Bottom 0.152: LED1.K 51.44,12.06 49.53,10.16 49.53,7.62 v48.26,6.35 | v41.91,5.08 41.91,3.81 40.64,2.54 17.78,2.54 16.51,3.81 16.51,10.16 10.79,15.88 7.62,15.88 6.35,17.14 6.35,18.41 S1.5
N$40  (via drill 0.3)
  Top 0.152: IC3.12 50.8,29.84 53.98,29.84 55.88,31.75 55.88,32.38 v58.42,32.38 | v63.5,39.37 63.5,41.91 68.58,46.99 68.58,48.26 69.22,48.9 77.47,48.9 81.28,45.09 91.44,45.09 92.08,44.45 v92.08,14.61 | v82.55,11.43 82.55,4.45 80.01,1.91 v61.59,1.91 | v48.9,1.91 8.26,1.91 1.27,8.89 1.27,34.29 R2.2
  Bottom 0.152: v58.42,32.38 58.42,33.02 60.96,35.56 61.59,35.56 63.5,37.47 v63.5,39.37 | v92.08,14.61 85.72,14.61 v82.55,11.43 | v48.9,1.91 v61.59,1.91
N$41  (via drill 0.3)
  Top 0.152: v14.61,31.11 15.88,29.84 17.14,31.11 17.14,32.38 20.95,36.2 33.02,36.2 v33.66,35.56 | v40.64,35.56 v36.83,35.56 | v43.18,35.56 43.81,34.92 45.09,34.92 48.9,38.73 IC3.3
  Bottom 0.152: IC2.5 19.05,37.47 19.05,36.83 14.61,32.38 v14.61,31.11 | v36.83,35.56 v33.66,35.56 | v43.18,35.56 v40.64,35.56
N$42  (via drill 0.3)
  Top 0.152: v29.84,22.23 v29.84,17.78 | v38.1,28.57 v48.26,28.57
  Bottom 0.152: EC1.33 27.94,15.88 v29.84,17.78 | v29.84,22.23 29.84,27.94 29.21,28.57 | IC2.12 29.21,28.57 | v48.26,28.57 IC3.13 | 29.21,28.57 v38.1,28.57
N$43
  Top 0.152: IC3.6 IC3.9
N$44  (via drill 0.3)
  Top 0.152: IC3.10 43.81,33.02 41.91,34.92 41.91,38.1 42.55,38.73 42.55,40.01 41.27,41.27 38.1,41.27 v37.47,40.64 | v35.56,42.55 35.56,46.35 34.92,46.99 v31.75,46.99
  Bottom 0.152: v35.56,42.55 v37.47,40.64 | v31.75,46.99 22.86,46.99 19.68,43.81 19.68,40.64 IC2.6
N$45
  Bottom 0.152: IC1.11 15.88,24.13 17.14,25.4 17.14,30.48 IC2.8
N$46  (via drill 0.3)
  Top 0.152: v19.05,27.94 v11.43,27.94 | v21.59,27.94 24.77,31.11 24.77,32.38 27.94,35.56 v30.48,35.56
  Bottom 0.152: S1.2 4.45,20.95 v11.43,27.94 | v21.59,27.94 v19.05,27.94 | v30.48,35.56 30.48,38.73 IC2.1
N$47  (via drill 0.3)
  Top 0.152: IC2.2 26.67,41.27 20.95,41.27 19.68,42.55 19.68,44.45 19.05,45.09 v19.05,46.99 | v19.05,48.26 19.05,50.16 IC5.6
  Bottom 0.152: v19.05,48.26 v19.05,46.99
N$48
  Top 0.152: IC2.11 IC2.10
N$49  (via drill 0.3)
  Top 0.152: v29.84,46.35 36.2,52.7 44.45,52.7 IC4.4
  Bottom 0.152: IC5.10 24.13,46.35 v29.84,46.35
N$50
  Bottom 0.152: IC5.4 25.4,52.7 33.66,52.7 43.18,43.18 IC4.10
N$51
  Top 0.152: IC5.8 13.97,45.09 13.97,45.72 6.35,45.72 JP1.1
N$52
  Bottom 0.152: IC5.5 18.41,53.34 12.7,53.34 8.26,48.9 8.26,44.45 JP2.2
N$53  (via drill 0.3)
  Top 0.152: v15.24,48.9 10.79,48.9 10.16,49.53 8.89,49.53 JP1.2
  Bottom 0.152: IC5.2 26.67,48.9 v15.24,48.9
N$54  (via drill 0.3)
  Top 0.152: v33.02,46.35 v33.02,40.64 | v13.34,45.09 6.35,45.09 JP2.1
  Bottom 0.152: IC3.8 34.92,31.75 33.02,33.66 v33.02,40.64 | v33.02,46.35 33.02,46.99 32.38,47.62 22.86,47.62 20.32,45.09 v13.34,45.09
N$55  (via drill 0.3)
  Top 0.152: IC1.19 36.2,21.59 32.38,25.4 32.38,29.84 v36.2,33.66 | v44.45,36.83 45.72,36.83 47.62,38.73 v47.62,42.55 | v65.41,45.09 v63.5,46.99
  Bottom 0.152: v36.2,33.66 36.83,33.66 40.01,36.83 v44.45,36.83 | v47.62,42.55 47.62,44.45 46.35,45.72 46.35,46.99 50.8,46.99 51.44,47.62 55.88,47.62 56.52,46.99 v63.5,46.99 | v65.41,45.09 67.94,45.09 D2.A
N$56  (via drill 0.3)
  Top 0.152: v28.57,20.95 IC1.16 | v16.51,20.95 9.53,27.94 9.53,31.11 15.88,37.47 v18.41,37.47 | v32.38,50.16 v27.94,45.72 | v36.2,48.9 38.73,48.9 v40.01,50.16 | v43.81,45.09 41.91,43.18 IC4.9
  Bottom 0.152: v16.51,20.95 v28.57,20.95 | v18.41,37.47 19.68,38.73 19.68,40.01 22.23,42.55 22.23,43.81 24.13,45.72 v27.94,45.72 | v32.38,50.16 33.66,50.16 34.29,49.53 35.56,49.53 v36.2,48.9 | v40.01,50.16 40.01,48.9 v43.81,45.09
N$57  (via drill 0.3)
  Top 0.152: D2.C D3.C | R4.2 13.34,31.11 19.68,37.47 33.02,37.47 IC4.8 41.27,45.72 v47.62,45.72
  Bottom 0.152: D2.C 60.33,43.81 59.69,43.18 56.52,43.18 53.98,45.72 v47.62,45.72
N$58  (via drill 0.3)
  Top 0.152: v60.33,19.68 IC6_PLCC.28 53.34,19.68 46.99,26.04 v41.27,26.04 | v70.48,19.05 67.94,19.05 66.67,20.32 v63.5,20.32
  Bottom 0.152: EC1.5 64.14,10.16 64.14,15.88 v60.33,19.68 60.33,23.5 61.59,23.5 63.5,21.59 v63.5,20.32 | IC2.13 30.48,29.84 38.1,29.84 41.27,26.67 v41.27,26.04 | IC6_DIL.28 71.12,18.41 v70.48,19.05
N$59  (via drill 0.3)
  Top 0.152: v36.2,32.38 IC1.2 | v42.55,36.2 42.55,34.92 43.18,34.29 45.72,34.29 50.16,38.73 50.16,40.01 51.44,41.27 v57.78,41.27 | D3.A v66.04,38.1
  Bottom 0.152: v36.2,32.38 40.01,36.2 v42.55,36.2 | v57.78,41.27 59.69,41.27 60.96,40.01 64.14,40.01 v66.04,38.1
VCC  (via drill 0.3)
  Top 0.152: C6.1 78.11,5.08 IC6_DIL.32 71.75,11.43 71.12,11.43 70.48,12.06 63.5,12.06 62.87,12.7 62.87,13.97 62.23,14.61 IC6_PLCC.32 62.23,19.05 60.96,20.32 53.34,20.32 49.53,24.13 49.53,25.4 C7.+ | IC4.14 56.52,45.72 C4.1 | IC3.14 56.52,34.29 C3.1 | 4.45,38.73 5.08,38.73 JP2.3 | 4.45,38.73 R3.1 | S1.4 7.62,24.13 1.91,29.84 1.91,32.38 R1.2 4.45,34.92 4.45,38.73 | IC2.14 33.66,34.29 C2.1 | v31.11,45.72 IC5.14 29.21,41.27 28.57,41.27 27.3,42.55 27.3,43.81 25.4,45.72 v19.68,45.72 | C1.1 39.37,18.41 IC1.20 | JP1.3 14.61,47.62 v16.51,45.72
  Bottom 0.152: IC3.14 49.53,27.3 49.53,25.4 C7.+ 48.9,25.4 47.62,24.13 43.18,24.13 41.91,25.4 | IC4.14 53.98,41.91 55.88,40.01 55.88,35.56 C3.1 | JP2.3 JP1.3 | IC5.14 31.11,41.27 29.84,40.01 29.84,33.02 IC2.14 32.38,31.75 33.66,30.48 38.1,30.48 41.91,26.67 41.91,25.4 | v31.11,45.72 C5.1 | EC1.27 35.56,15.24 IC1.20 | 41.91,25.4 40.64,24.13 40.64,22.23 C1.1 | v19.68,45.72 v16.51,45.72

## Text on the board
tNames: MEGAFLASH WILCO2009 / INITIAL DESIGN BY BRYCE | OFF | ON | OFF | READ | WRITE
bNames: MEGAFLASH WILCO2009 / INITIAL DESIGN BY BRYCE
tValues: ON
